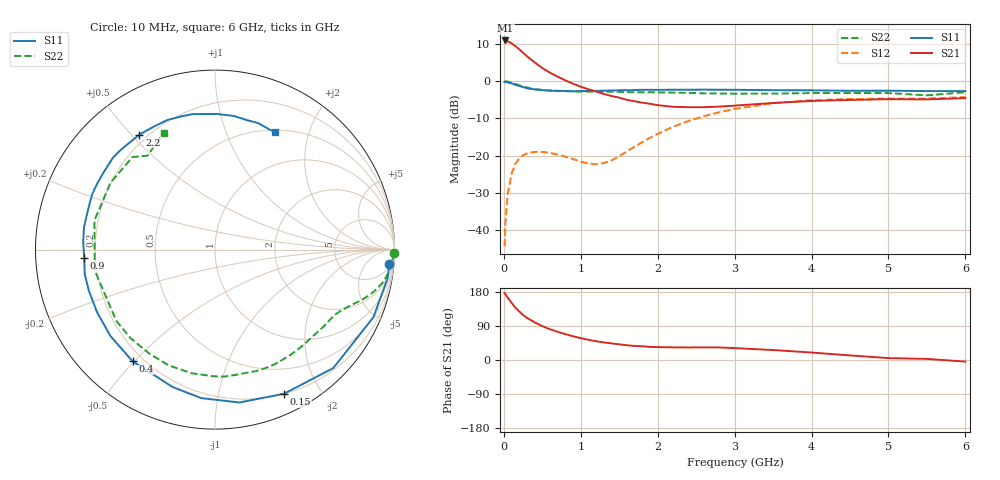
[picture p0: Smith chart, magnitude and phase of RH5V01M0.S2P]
! SIEMENS Small Signal Semiconductors
! BFR106
! Si NPN RF Bipolar Junction Transistor in SOT23
! VCE = 5 V  IC = 1 mA
! Common Emitter S-Parameters:  August  1996
# GHz  S  MA  R  50
!  f  S11  S21  S12  S22
! GHz  MAG  ANG  MAG  ANG  MAG  ANG  MAG  ANG
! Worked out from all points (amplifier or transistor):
!   36 points, 10 MHz to 6 GHz, reference 50 ohm
!   highest |S21| = 10.9 dB at 20 MHz (marker M1)
!   |S21| within 3 dB of that: start of sweep to 234.3 MHz
!   unconditionally stable (mu >= 1): 857.4 MHz to 2.003 GHz; 2.713 GHz to end of sweep
!   at 250 MHz: K = 0.26, MSG = 13.7 dB, |S12| = -19.9 dB
!   at 1.4 GHz: K = 1.43, MAG = 4.8 dB, |S12| = -21.3 dB
!   at 6 GHz: K = 1.02, MAG = -0.9 dB, |S12| = -4.3 dB
!   S11 on the Smith chart (normalised r, x): 10 MHz: 7, -22; 150 MHz: 0.20, -1.57; 400 MHz: 0.16, -0.49; 900 MHz: 0.16, -0.03; 2.2 GHz: 0.17, +0.53; 6 GHz: 0.53, +1.51
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0.01  0.9739 -4.8  3.507 176.3  0.0061 88.9  1 -1.2
0.02  0.9749 -9.4  3.513 174.0  0.0121 86.3  0.9927 -2.3
0.05  0.9597 -23.1  3.424 164.4  0.0306 76.7  0.9854 -5.6
0.1  0.9328 -45.0  3.22 151.3  0.0572 65.6  0.9571 -10.7
0.15  0.8904 -64.4  2.948 138.0  0.0775 54.3  0.9171 -14.7
0.2  0.8627 -80.9  2.681 128.1  0.0915 46.3  0.8805 -17.7
0.25  0.831 -95.3  2.403 118.7  0.1014 39.0  0.8473 -20.1
0.3  0.8013 -107.1  2.157 111.4  0.1072 34.3  0.8228 -21.9
0.4  0.7736 -126.4  1.788 99.4  0.1123 26.0  0.7845 -25.3
0.5  0.7557 -140.5  1.498 89.4  0.112 20.9  0.7617 -28.3
0.6  0.7439 -152.0  1.297 81.1  0.1089 18.0  0.7499 -31.5
0.9  0.73 -176.2  0.922 62.7  0.0901 19.9  0.7274 -42.1
1.1  0.7402 170.4  0.778 53.3  0.0783 31.5  0.7233 -50.0
1.3  0.7442 159.9  0.671 46.4  0.0796 50.5  0.7197 -58.3
1.6  0.754 146.6  0.561 38.9  0.1139 72.4  0.7142 -71.5
2.2  0.7667 123.3  0.452 33.4  0.2442 75.0  0.7009 -100.9
2.8  0.7656 104.5  0.455 33.1  0.3825 60.7  0.6819 -133.7
3.5  0.756 89.2  0.509 26.3  0.506 41.8  0.6802 -170.2
4.5  0.7428 76.0  0.559 12.1  0.5745 18.4  0.6914 147.3
5  0.7448 71.2  0.572 5.0  0.5838 9.7  0.6909 131.7
5.5  0.735 65.8  0.568 2.9  0.5832 5.6  0.6443 125.7
6  0.7353 62.8  0.592 -4.3  0.6095 -2.5  0.7101 113.8
